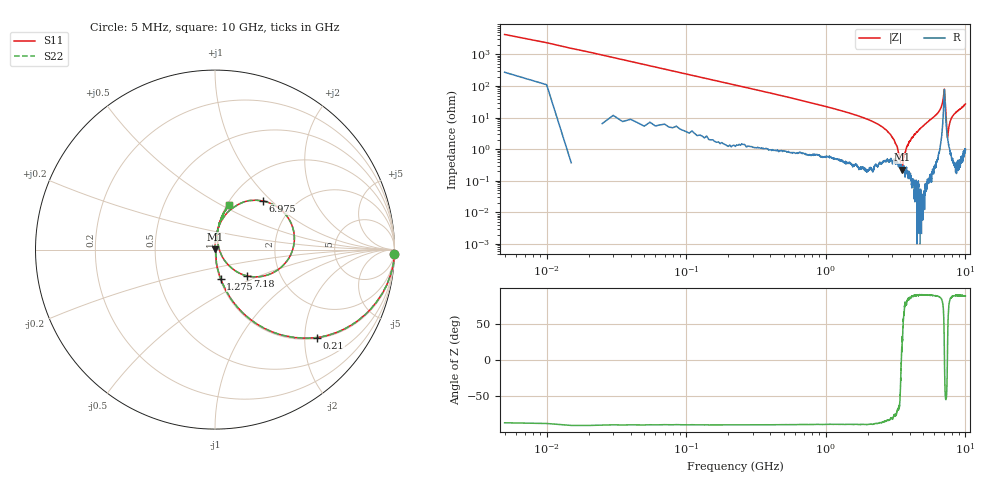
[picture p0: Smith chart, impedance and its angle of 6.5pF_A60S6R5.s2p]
! Amotech Co.,Ltd.
! http://www.amotech.co.kr/
! Part Number: A60S6R5
! These Parameters are Measured in Series Mode Connection
! Operation Temp=25[degC], DC Bias Voltage=0[V]
! Freq. Start=5[MHz] Stop=10[GHz], 2000[Steps]
! Date: Monday, July 13, 2020, 01:56:27
# GHZ S RI R 50.000000
!Freq.(Hz) S11(Real) S11(Imag) S21(Real) S21(Imag) S12(Real) S12(Imag) S22(Real) S22(Imag)
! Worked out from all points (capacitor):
!   2000 points, 5 MHz to 10 GHz, reference 50 ohm
!   read as one part in series: C = 6.62 pF near 55 MHz
!   lowest |Z| = 225 mohm at 3.535 GHz (marker M1)
!   series resonance near 3.476 GHz, so ESL is about 320 pH
!   S11 on the Smith chart (normalised r, x): 5 MHz: 6, -85; 210 MHz: 1.02, -2.30; 1.275 GHz: 1.01, -0.34; 6.975 GHz: 1.40, +0.89; 7.18 GHz: 1.36, -0.42; 10 GHz: 1.02, +0.54
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0.005  0.998 -0.0232  0.00203 0.0232  0.00203 0.0232  0.998 -0.0232
0.085  0.8841 -0.3108  0.1159 0.3108  0.1159 0.3108  0.8841 -0.3108
0.21  0.5691 -0.49  0.4309 0.49  0.4309 0.49  0.5691 -0.49
0.55  0.1617 -0.359  0.8383 0.359  0.8383 0.359  0.1617 -0.359
1.275  0.0314 -0.162  0.9686 0.162  0.9686 0.162  0.0314 -0.162
1.675  0.0165 -0.1144  0.9835 0.1144  0.9835 0.1144  0.0165 -0.1144
2.855  0.00525 -0.0313  0.9948 0.0313  0.9948 0.0313  0.00525 -0.0313
3.205  0.00363 -0.0128  0.9964 0.0128  0.9964 0.0128  0.00363 -0.0128
3.34  0.00318 -0.00627  0.9968 0.00627  0.9968 0.00627  0.00318 -0.00627
3.485  0.00268 0.000182  0.9973 -0.000182  0.9973 -0.000182  0.00268 0.000182
3.535  0.00203 0.000951  0.998 -0.000951  0.998 -0.000951  0.00203 0.000951
3.65  0.00252 0.00642  0.9975 -0.00642  0.9975 -0.00642  0.00252 0.00642
3.965  0.00149 0.0172  0.9985 -0.0172  0.9985 -0.0172  0.00149 0.0172
5.005  0.00322 0.0556  0.9968 -0.0556  0.9968 -0.0556  0.00322 0.0556
6.67  0.053 0.1867  0.947 -0.1867  0.947 -0.1867  0.053 0.1867
6.975  0.2685 0.2708  0.7315 -0.2708  0.7315 -0.2708  0.2685 0.2708
7.07  0.4419 0.0463  0.5581 -0.0463  0.5581 -0.0463  0.4419 0.0463
7.18  0.1787 -0.1468  0.8213 0.1468  0.8213 0.1468  0.1787 -0.1468
7.45  0.0217 0.00738  0.9783 -0.00738  0.9783 -0.00738  0.0217 0.00738
7.77  0.0134 0.0731  0.9866 -0.0731  0.9866 -0.0731  0.0134 0.0731
8.335  0.0195 0.1274  0.9805 -0.1274  0.9805 -0.1274  0.0195 0.1274
10  0.076 0.2479  0.924 -0.2479  0.924 -0.2479  0.076 0.2479
